(*  *)
PROGRAM MAIN
VAR
	(* EL1918 做主逻辑与 AMP8000 通讯时，若 AMP8000 的复位信号
	由 EL1918传递过来，且两者都有报警，给的复位信号需要给2次，
	因为第一次是复位 EL1918的，第二次才能复位 AMP8000 的，即
	逻辑报警时不会 FSOE 不会传输数据
	*)
	EL1918Control	:	FB_SAFE_CONTROL;
	//AMP_5Control	:	FB_SAFE_CONTROL;
	
	
END_VAR

arAxis[1]();
arAxis[2]();
arAxis[3]();
arAxis[4]();
arAxis[5]();

EL1918Control();

END_PROGRAM
